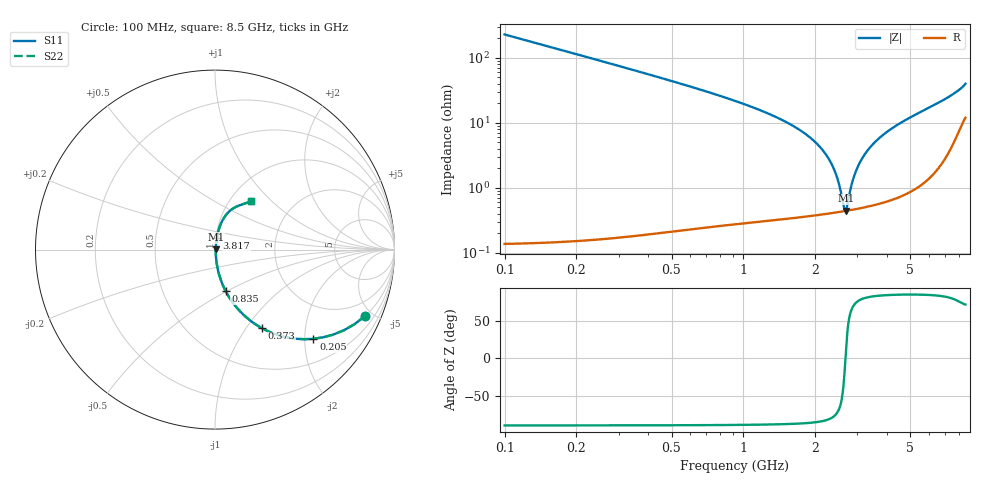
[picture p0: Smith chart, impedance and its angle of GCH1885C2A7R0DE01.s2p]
!Murata Part Number: GCH1885C2A7R0DE01
!These Parameters are Measured in Series Mode Connection
!Data Generated on Mar 13, 2026
!  o--ll--o
!Port1  Port2
!  o------o
!Operation Temp=25[degC], DC Bias Voltage=0[V]
!Freq. Start=100[MHz] Stop=9[GHz] 401[Steps]
# Hz S RI R 50
!Freq.(Hz) S11(Real) S11(Imag) S21(Real) S21(Imag) S12(Real) S12(Imag) S22(Real) S22(Imag)
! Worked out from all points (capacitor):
!   401 points, 100 MHz to 8.5 GHz, reference 50 ohm
!   read as one part in series: C = 7 pF near 142 MHz
!   lowest |Z| = 446 mohm at 2.683 GHz (marker M1)
!   series resonance near 2.674 GHz, so ESL is about 510 pH
!   S11 on the Smith chart (normalised r, x): 100 MHz: 1.00, -4.54; 205 MHz: 1.00, -2.20; 373 MHz: 1.00, -1.19; 835 MHz: 1.01, -0.49; 3.817 GHz: 1.01, +0.13; 8.5 GHz: 1.24, +0.76
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1e8  0.8373 -0.3687  0.1627 0.3687  0.1627 0.3687  0.8373 -0.3687
2.05e8  0.5484 -0.497  0.4516 0.497  0.4516 0.497  0.5484 -0.497
2.89e8  0.3767 -0.4835  0.6233 0.4835  0.6233 0.4835  0.3767 -0.4835
3.73e8  0.2635 -0.4389  0.7365 0.4389  0.7365 0.4389  0.2635 -0.4389
5.62e8  0.1311 -0.3347  0.8689 0.3347  0.8689 0.3347  0.1311 -0.3347
8.35e8  0.0589 -0.2302  0.9411 0.2302  0.9411 0.2302  0.0589 -0.2302
1.507e9  0.0137 -0.1011  0.9863 0.1011  0.9863 0.1011  0.0137 -0.1011
1.969e9  0.00649 -0.0524  0.9935 0.0524  0.9935 0.0524  0.00649 -0.0524
2.263e9  0.00481 -0.0284  0.9952 0.0284  0.9952 0.0284  0.00481 -0.0284
2.452e9  0.00439 -0.0147  0.9956 0.0147  0.9956 0.0147  0.00439 -0.0147
2.641e9  0.00437 -0.00209  0.9956 0.00209  0.9956 0.00209  0.00437 -0.00209
2.683e9  0.0044 0.000592  0.9956 -0.000592  0.9956 -0.000592  0.0044 0.000592
2.725e9  0.00446 0.00323  0.9955 -0.00323  0.9955 -0.00323  0.00446 0.00323
2.83e9  0.00465 0.00968  0.9953 -0.00968  0.9953 -0.00968  0.00465 0.00968
2.914e9  0.00486 0.0147  0.9951 -0.0147  0.9951 -0.0147  0.00486 0.0147
3.061e9  0.00535 0.0231  0.9947 -0.0231  0.9947 -0.0231  0.00535 0.0231
3.25e9  0.00617 0.0336  0.9938 -0.0336  0.9938 -0.0336  0.00617 0.0336
3.817e9  0.00977 0.0625  0.9902 -0.0625  0.9902 -0.0625  0.00977 0.0625
4.3e9  0.0141 0.0854  0.9859 -0.0854  0.9859 -0.0854  0.0141 0.0854
5.707e9  0.0346 0.1483  0.9654 -0.1483  0.9654 -0.1483  0.0346 0.1483
7.114e9  0.0794 0.2127  0.9206 -0.2127  0.9206 -0.2127  0.0794 0.2127
8.5e9  0.1984 0.2714  0.8016 -0.2714  0.8016 -0.2714  0.1984 0.2714
